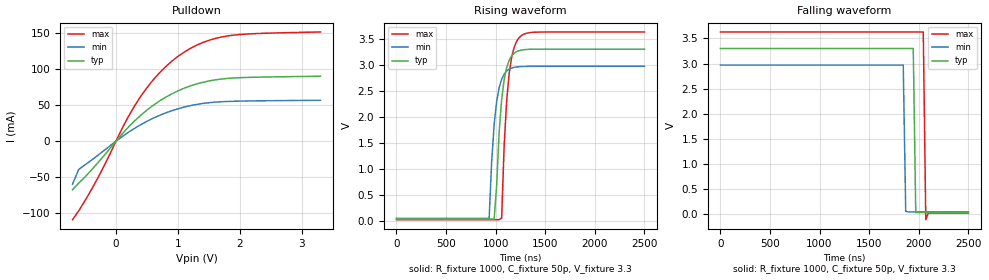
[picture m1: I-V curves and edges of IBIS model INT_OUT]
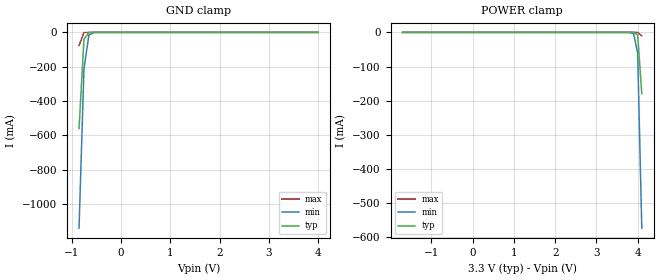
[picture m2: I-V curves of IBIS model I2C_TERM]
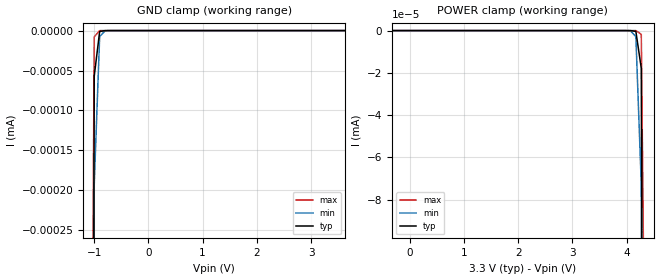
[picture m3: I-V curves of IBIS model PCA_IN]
|   NXP Semiconductors Inc.
|   Specialty Logic Products Group
|   IBIS model of PCA9543C
|   2-Channel I2C switch with
|   interrupt logic and reset
[IBIS Ver]   3.2
[Comment Char]   |_char
|  VDD: Typ: 3.3v, Min: 2.97v, 3.3v
[File name]   pca9543c_3_3v.ibs
[File Rev]   1.0
[Date]   Dec 12, 2007 11:20:50 AM
[Source]
Generated by Seshadri Venkataramanan with IbisToolKit at Tempe, AZ
[Notes]
[Disclaimer]
(C) Copyright 2007 NXP Semiconductors
All rights reserved
NXP Semiconductors (NXP) does not warrant that this model and any other
accompanying information (Model) accurately or fully represents the
operating characteristics and specifications of the semiconductor
products to which the Model relates.  Moreover, the Model is furnished
on an "as is" and with "all faults" basis, and without support or
warranty of any kind.  NXP disclaims all warranties, whether expressed
or implied or statutory, including without limitation all implied
warranties of non-infringement, merchantability and fitness for any
purpose, and those arising from a course of dealing or usage of trade.
NXP does not convey any license under its or any third party's patents,
copyrights or other intellectual property or proprietary rights.
You and your company assume any and all risks and liability arising out
of the application or use of the Model.
In no event shall NXP be liable for any direct, indirect, special,
consequential or incidental damages, however caused, whether in
warranty, contract or tort (including negligence), strict liability or
other legal theory, including, without limitation, for lost profits,
business interruption, or corruption or loss of data or information,
arising out of or in connection with the use of or the inability to use
the Model, even if NXP has been advised of the possibility of such
damages.
NXP provides the Model as a courtesy to our customers. You and your
company shall not distribute, convey, sell, or give the Model to anyone
else without receiving prior written permission from NXP.
NXP reserves the right to make changes without notice to the Model to
improve reliability, function, or design.
Please be aware that your receipt and subsequent use of the Model shall
serve as acceptance of these terms and conditions.  If you do not
accept these terms, return or destroy the Model immediately.
[Copyright]
2007
[Component]   PCA9543AD
Si_location Pin
Timing_location Pin
[Manufacturer]   NXP Semiconductors
[Package]
|   variable   typ   min   max
R_pkg   4.54E-02   4.38E-02   5.01E-02
L_pkg   2.31E-09   1.63E-09   3.26E-09
C_pkg   0.565E-12   0.437E-12   0.736E-12
|   SO14
[Pin] signal_name   model_name   R_pin   L_pin   C_pin
1   A0   PCA_IN   4.18E-02  3.26E-09  0.675E-12
2   A1   PCA_IN   5.01E-02  2.30E-09  0.574E-12
3   RESETB   PCA_IN   4.52E-02  1.71E-09  0.467E-12
4   INT0B   INT_IN   4.38E-02  1.63E-09  0.437E-12
5   SD0   I2C_TERM   4.52E-02  1.71E-09  0.465E-12
6   SC0   I2C_TERM   5.01E-02  2.30E-09  0.573E-12
7   VSS   GND   4.18E-02  3.26E-09  0.736E-12
8   INT1B   INT_IN   4.18E-02  3.26E-09  0.736E-12
9   SD1   I2C_TERM   5.01E-02  2.30E-09  0.573E-12
10   SC1   I2C_TERM   4.52E-02  1.71E-09  0.465E-12
11   INTB   INT_OUT   4.38E-02  1.63E-09  0.437E-12
12   SCL   I2C_TERM   4.52E-02  1.71E-09  0.467E-12
13   SDA   I2C_TERM   5.01E-02  2.30E-09  0.574E-12
14   VDD   POWER   4.18E-02  3.26E-09  0.736E-12
[Component]   PCA9543APW
Si_location Pin
Timing_location Pin
[Manufacturer]   NXP Semiconductors
[Package]
|   variable   typ   min   max
R_pkg   3.44E-02   2.80E-02   4.33E-02
L_pkg   1.83E-09   1.36E-09   2.32E-09
C_pkg   0.380E-12   0.302E-12   0.442E-12
|   TSSOP14
[Pin] signal_name   model_name   R_pin   L_pin   C_pin
1   A0   PCA_IN   3.46E-02  2.32E-09  0.423E-12
2   A1   PCA_IN   4.33E-02  2.04E-09  0.441E-12
3   RESETB   PCA_IN   2.80E-02  1.36E-09  0.307E-12
4   INT0B   INT_IN   2.88E-02  1.38E-09  0.302E-12
5   SD0   I2C_TERM   2.80E-02  1.36E-09  0.308E-12
6   SC0   I2C_TERM   4.33E-02  2.04E-09  0.441E-12
7   VSS   GND   3.46E-02  2.32E-09  0.433E-12
8   INT1B   INT_IN   3.46E-02  2.32E-09  0.433E-12
9   SD1   I2C_TERM   4.33E-02  2.04E-09  0.441E-12
10   SC1   I2C_TERM   2.80E-02  1.36E-09  0.308E-12
11   INTB   INT_OUT   2.88E-02  1.38E-09  0.302E-12
12   SCL   I2C_TERM   2.80E-02  1.36E-09  0.308E-12
13   SDA   I2C_TERM   4.33E-02  2.04E-09  0.442E-12
14   VDD   POWER   3.46E-02  2.31E-09  0.433E-12
[Series Pin Mapping] pin_2 model_name   function_table_group
5   13   PCA_SW   1
6   12   PCA_SW   1
9   13   PCA_SW   2
10   12   PCA_SW   2
[Series Switch Groups]
|   Default both off
Off 1 2 /
|   Other possibilities
On 1 /
On 2 /
[Model]   PCA_SW
Model_type Series_switch
C_comp   0.5p   0.5p   0.5p
[Temperature Range] 27   -40   85
[Voltage Range]   3.3   2.3   5.5
[Pullup Reference]  3.3   2.3   5.5
[Pulldown Reference]0   0   0
[On]
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[Off]
|   variable   R(typ)   R(min)   R(max)
[R Series]   1e06   1e06   1e06
|[End   PCA_SW
| Models and submodels in the file (5): INT_OUT (Open_drain), I2C_TERM (Terminator), PCA_IN (Input), INT_IN (Input), PCA_SW (Series_switch)
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[Model]   INT_OUT
Model_type Open_drain
Vref=3.3
Vmeas=1.65
Rref=1000
Cref=1p
C_comp   2.2p   2p   2.3p
[Model Spec]
Vmeas   1.65   1.485   1.815
[Temperature Range] 27   85   -40
[Voltage Range]   3.3   2.97   3.63
[Pullup Reference]  3.3   2.97   3.63
[Pulldown Reference]0   0   0
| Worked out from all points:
|   slope of the pulldown table from 0 to 0.495 V, typ, clamps not added: 11.6 ohm
|   falling waveform, R_fixture 1000, C_fixture 50p, V_fixture 3.3: 20-80 % time 15.2ns typ, 15.2ns min, 14.6ns max; typ from 3.3 V to 0.031 V
|   rising waveform, R_fixture 1000, C_fixture 50p, V_fixture 3.3: 20-80 % time 71ns typ, 70.9ns min, 69.5ns max; typ from 0.031 V to 3.3 V
[Pulldown]
-700mV    -67.14mA   -59.47mA   -108.7mA
-600mV    -57.94mA   -39.06mA   -96.38mA
-300mV    -30.61mA   -20.02mA   -52.1mA
100mV     10.13mA    6.387mA    17.87mA
300mV     28.11mA    17.87mA    48.86mA
600mV     49.71mA    31.88mA    84.94mA
800mV     60.9mA     39.19mA    103.2mA
1V        69.82mA    44.98mA    117.6mA
1.4V      81.7mA     52.36mA    136.8mA
1.8V      87.05mA    55.15mA    146mA
2.2V      88.63mA    55.9mA     149mA
3.3V      90.08mA    56.79mA    151.4mA
[Falling Waveform]
R_fixture=1000
C_fixture=50p
V_fixture=3.3
V_fixture_min=2.97
V_fixture_max=3.63
0s        3.3V       2.97V      3.63V
1.843us   3.3V       2.97V      3.63V
1.869us   3.3V       55.63mV    3.63V
1.944us   3.3V       45.02mV    3.63V
1.97us    31.91mV    45.02mV    3.63V
2.045us   31.49mV    45.02mV    3.63V
2.071us   31.49mV    45.02mV    -110.4mV
2.096us   31.48mV    45.03mV    19.53mV
2.5us     31.48mV    45.02mV    19.53mV
[Rising Waveform]
R_fixture=1000
C_fixture=50p
V_fixture=3.3
V_fixture_min=2.97
V_fixture_max=3.63
0s        31.48mV    45.02mV    19.53mV
934.3ns   31.5mV     46.79mV    19.55mV
959.6ns   31.49mV    1.13V      19.55mV
984.8ns   31.5mV     1.853V     19.55mV
1.061us   2.336V     2.721V     52.47mV
1.086us   2.716V     2.819V     1.454V
1.136us   3.085V     2.914V     2.831V
1.187us   3.221V     2.95V      3.337V
1.263us   3.282V     2.965V     3.565V
2.5us     3.3V       2.97V      3.63V
[Ramp]
R_load=1000
dV/dt_r   1.961E+0/8.946E-10   1.950E+0/1.230E-9   1.969E+0/1.178E-9
dV/dt_f   1.961E+0/1.225E-9   1.950E+0/1.510E-9   1.969E+0/7.190E-10
|[End   INT_OUT
| [End   I2C_TERM
|  [End   I2C_TERM
[Model]   I2C_TERM
Model_type Terminator
C_comp   9.5p   9.5p   9.5p
[Temperature Range] 27   85   -40
[Voltage Range]   3.3   2.97   3.63
[Pullup Reference]  3.3   2.97   3.63
[Pulldown Reference]0   0   0
[POWER Clamp Reference]3.3   2.97   3.63
[GND Clamp Reference]0   0   0
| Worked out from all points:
|   GND clamp passes 1 mA (typ) near -0.62 V on its own axis
[GND Clamp]
|   -6.000000E-1   -1.554225E-1   -1.242642E-1   -2.666059E-1
|   -5.000000E-1   -1.602113E-1   -1.179351E-1   -2.662641E-1
|   -4.000000E-1   -1.574088E-1   -1.099432E-1   -2.800035E-1
-850mV    -559.4mA   -1.139A    -76.35mA
-750mV    -40.51mA   -212.7mA   -980.8uA
-650mV    -1.325mA   -15.66mA   -6.907uA
-550mV    -28.76uA   -821uA     -47.66nA
-450mV    -602.7nA   -33.06uA   -372.7pA
4V        327pA      361.9pA    339.8pA
[POWER Clamp]
-1.7V     378pA      421.6pA    390.2pA
3.7V      -87.23nA   -6.548uA   -66.84pA
3.8V      -4.165uA   -166.2uA   -4.002nA
3.9V      -197.8uA   -3.8mA     -573.6nA
4V        -7.959mA   -60.35mA   -83.06uA
4.1V      -179.8mA   -573.3mA   -10.08mA
[Model]   PCA_IN
Model_type Input
Vinh=2.1
Vinl=0.9
C_comp   1.73p   1.73p   1.73p
[Temperature Range] 27   85   -40
[Voltage Range]   3.3   2.97   3.63
[POWER Clamp Reference]3.3   2.97   3.63
[GND Clamp Reference]0   0   0
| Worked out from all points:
|   GND clamp passes 1 mA (typ) near -1.21 V on its own axis
[GND Clamp]
-2V       -10.17A    -9.093A    -11.52A
-1.1V     -2.718uA   -4.916uA   -1.14uA
-1V       -56.9nA    -192.5nA   -7.858nA
-900mV    -1.192nA   -7.538nA   -55.05pA
-800mV    -25.74pA   -295.9pA   -1.173pA
-700mV    -1.222pA   -12.26pA   -702.6fA
3.63V     3.63pA     3.63pA     3.63pA
[POWER Clamp]
-330mV    3.63pA     3.63pA     3.63pA
3.97V     -833.7fA   -5.042pA   -670.6fA
4.07V     -8.589pA   -112.4pA   -853.8fA
4.17V     -374.3pA   -2.852nA   -13.03pA
4.27V     -17.84nA   -72.82nA   -1.766nA
4.37V     -852.2nA   -1.86uA    -256.1nA
5.27V     -9.601A    -8.532A    -10.94A
